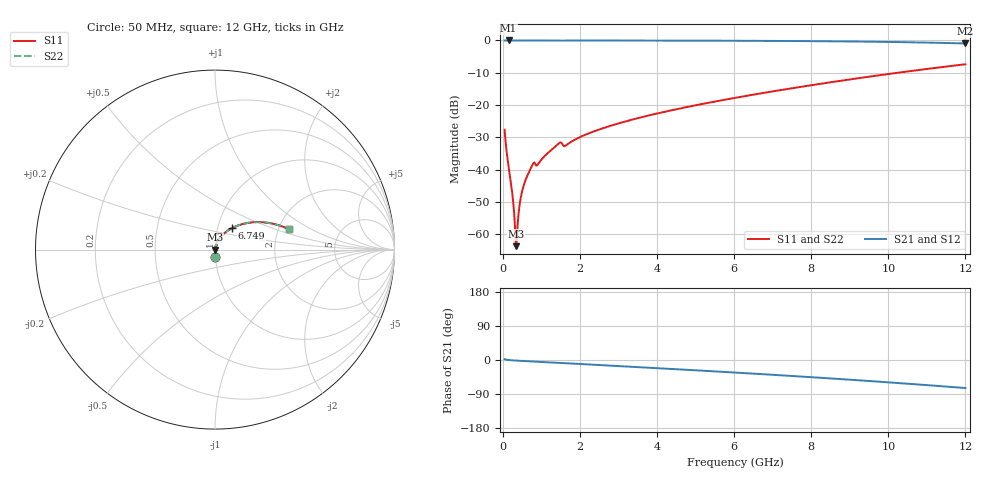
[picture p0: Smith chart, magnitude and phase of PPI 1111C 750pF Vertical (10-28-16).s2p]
# GHz S MA R 50
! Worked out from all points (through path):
!   1601 points, 50 MHz to 12 GHz, reference 50 ohm
!   highest |S21| = 0.00 dB at 154.6 MHz (marker M1); lowest = -0.9 dB at 12 GHz (marker M2)
!   group delay of S21, straight-line fit = 16.9 ps
!   lowest |S11| = -63.7 dB at 348.8 MHz (marker M3), VSWR 1.00, Z = 50.1 - j0.00877 ohm
!   |S11| at or under -10 dB: start of sweep to 10.24 GHz
!   |S22| runs from -63.7 to -7.4 dB; largest |S21 - S12| = 0
!   S11 on the Smith chart (normalised r, x): 50 MHz: 1.00, -0.08; 6.749 GHz: 1.17, +0.29; 12 GHz: 2.28, +0.63
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0.05  0.04151 -87.4  0.9988 2.2  0.9988 2.2  0.04151 -87.4
0.08734375  0.02277 -88.1  0.9994 0.9  0.9994 0.9  0.02277 -88.1
0.1545625  0.01108 -87.6  0.9995 -0.0  0.9995 -0.0  0.01108 -87.6
0.2441875  0.004525 -83.7  0.9994 -0.8  0.9994 -0.8  0.004525 -83.7
0.3114062  0.001578 -68.1  0.9994 -1.3  0.9994 -1.3  0.001578 -68.1
0.34875  0.0006558 -7.7  0.9993 -1.5  0.9993 -1.5  0.0006558 -7.7
0.3860938  0.001357 58.1  0.9993 -1.8  0.9993 -1.8  0.001357 58.1
0.4533125  0.003264 74.8  0.9992 -2.2  0.9992 -2.2  0.003264 74.8
0.528  0.005258 78.7  0.9992 -2.6  0.9992 -2.6  0.005258 78.7
0.6250938  0.007726 80.1  0.999 -3.2  0.999 -3.2  0.007726 80.1
0.7744688  0.01193 77.4  0.9981 -4.1  0.9981 -4.1  0.01193 77.4
0.916375  0.01218 76.1  0.9979 -4.7  0.9979 -4.7  0.01218 76.1
1.454125  0.02556 74.8  0.9963 -7.8  0.9963 -7.8  0.02556 74.8
1.633375  0.02355 73.0  0.9961 -8.4  0.9961 -8.4  0.02355 73.0
2.044156  0.03275 76.4  0.9977 -10.8  0.9977 -10.8  0.03275 76.4
2.873187  0.04934 72.7  0.9969 -15.3  0.9969 -15.3  0.04934 72.7
4.038312  0.07483 66.7  0.9949 -21.7  0.9949 -21.7  0.07483 66.7
6.025  0.1292 55.7  0.9887 -33.1  0.9887 -33.1  0.1292 55.7
6.749469  0.1536 51.5  0.9849 -37.5  0.9849 -37.5  0.1536 51.5
8.019156  0.2035 43.7  0.9753 -45.4  0.9753 -45.4  0.2035 43.7
10.01331  0.303 30.2  0.9484 -59.0  0.9484 -59.0  0.303 30.2
12  0.4279 15.3  0.8981 -74.0  0.8981 -74.0  0.4279 15.3
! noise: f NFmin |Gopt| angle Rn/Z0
0.05  0.0003805  0.8688  0.2419  0.0006239
1.372  0.004957  0.7428  5.919  0.003858
2.701  0.006689  0.6475  11.47  0.003565
4.031  0.00895  0.6178  16.87  0.004273
5.36  0.01118  0.6026  22.11  0.005012
6.682  0.01343  0.596  27.14  0.005792
8.012  0.01577  0.5961  32.01  0.006663
9.341  0.01826  0.6016  36.69  0.007668
10.67  0.02098  0.612  41.2  0.008866
12  0.02401  0.6266  45.56  0.01033
